| IBIS file generated by GenIBIS.pl Version 3.28
|   awr1642_q1_3v3_fcbga161
[IBIS ver]   4.1
[File name]   awr1642_q1_3v3_fcbga161.ibs
[File Rev]   1.1
[Date]   Mon Mar 13, 2017, 18:0:35
[Source]   Data created at Texas Instruments
[Notes]   1) NOT YET CHECKED BY IBISCK4. Once checked update notes
   section with any relevant information.
   2) Model not valid until this section updated.
   Some pins may contain selectors which are not valid options
   for that particular pin.
   Please refer to the device datasheet for information on picking
   the correct selector model, which depends on various software
   register configurations.
   Some pins are modeled as IO or tri-state for output mode.
   3) converted rev1.0 to rev1.1 by hand, part# change
[Disclaimer] Please be aware that in the absence of a written agreement,
   Texas Instruments (TI) assumes no liability for: 1) the
   accuracy of the IBIS models provided to your company, 2) the
   proper functioning of these IBIS models in your design or for
   any resulting applications, or, 3) infringement of patents,
   copyrights, or intellectual property rights resulting from
   your use of these IBIS models. TI provides IBIS models as a
   service to our customers and therefore reserves the right to
   limit distribution of the IBIS models.
[Copyright]   Property of Texas Instruments Incorporated. Unauthorised
   reproduction and/or distribution is strictly prohibited. This
   product is protected under copyright law and trade secret law
   as an unpublished work. Created 2010,(C) Copyright 2010,
   Texas Instruments Incorporated., All Rights Reserved. These
   commodities are under the U.S. Government distribution license
   control.As such,they are not to be re-exported without the
   prior approval of the U.S. Department of Commerce.
|   Component awr1642_q1_3v3_fcbga161
[Component]   awr1642_q1_3v3_fcbga161
[Manufacturer]   Texas Instruments.
| Source IO level model revisions
|Model   Revision   Date
|BC1833DV40DCPBFBP18LL_OD_FS_SSDLV  1.0   May 27, 2010
|OLVDS18_SSDHH   1.0   Nov 14, 2016
|BC1833DV40DCPBFBP18LL_SSDLV   1.0   May 27, 2010
[Package Model] awr1642_q1_3v3_fcbga161
[Package]
|   typ   min   max
R_pkg   0.147827121052632   18.2775E-3   506.793E-3
L_pkg   1.74484056140351E-009 0.245382E-9   5.35555E-9
C_pkg   7.81909035087719E-013 0.285311E-12   2.03823E-12
[Pin]   signal_name   model_name
D15   CLKM   NC
C15   CLKP   NC
P1   GPADC_1   NC
B13   GPADC_5   NC
P2   GPADC_2   NC
R2   GPADC_4   NC
P3   GPADC_3   NC
C14   GPADC_6   NC
H13   GPIO_0   Selector_3
J13   GPIO_1   Selector_3
K13   GPIO_2   Selector_3
K14   LVDS_TXP[1]   Model_25
J14   LVDS_TXP[0]   Model_25
L15   LVDS_CLKM   Model_25
M15   LVDS_FRCLKM   Model_25
M14   LVDS_FRCLKP   Model_25
K15   LVDS_TXM[1]   Model_25
J15   LVDS_TXM[0]   Model_25
L14   LVDS_CLKP   Model_25
N8   MCU_CLKOUT   Selector_1
N7   NERROR_IN   Selector_2
N6   NERROR_OUT   Selector_5
R3   NRESET   NC
A14   OSC_CLKOUT   NC
P9   PMIC_CLKOUT   Selector_1
N12   QSPI[1]   Selector_3
R14   QSPI[2]   Selector_3
R12   QSPI_CLK   Selector_1
R13   QSPI[0]   Selector_3
P12   QSPI[3]   Selector_3
P11   QSPI_CS_N   Selector_1
N4   RS232_RX   Selector_6
N5   RS232_TX   Selector_1
M2   RX1   NC
K2   RX2   NC
H2   RX3   NC
F2   RX4   NC
P13   SPI_HOST_INTR   Selector_1
E14   SPIA_MISO   Selector_1
D13   SPIA_MOSI   Selector_6
C13   SPIA_CS_N   Selector_6
E13   SPIA_CLK   Selector_6
F13   SPIB_MOSI   Selector_6
H14   SPIB_CS_N   Selector_6
G14   SPIB_MISO   Selector_1
F14   SPIB_CLK   Selector_6
P4   SYNC_IN   Selector_6
G13   SYNC_OUT   Selector_1
P10   TCK   Selector_6
R11   TDI   Selector_6
N13   TDO   Selector_1
N10   TMS   Selector_6
B8   TRACE_DATA_14   Selector_6
N15   TRACE_CLK   Selector_6
C9   TRACE_DATA_11   Selector_6
P6   TRACE_DATA_3   Selector_6
P5   TRACE_DATA_1   Selector_6
C8   TRACE_DATA_12   Selector_6
B14   TRACE_DATA_9   Selector_6
R4   TRACE_DATA_0   Selector_6
P8   TRACE_DATA_7   Selector_6
P7   TRACE_DATA_5   Selector_6
R5   TRACE_DATA_2   Selector_6
N14   TRACE_CTL   Selector_6
A9   TRACE_DATA_15   Selector_6
R8   TRACE_DATA_6   Selector_6
R7   TRACE_DATA_4   Selector_6
B9   TRACE_DATA_13   Selector_6
B15   TRACE_DATA_10   Selector_6
D14   TRACE_DATA_8   Selector_6
B4   TX1   NC
B6   TX2   NC
B10   VBGAP   NC
H15   VDDIN   NC
N11   VDDIN   NC
P15   VDDIN   NC
R6   VDDIN   NC
C2   VIN_13RF2   NC
D2   VIN_13RF2   NC
F5   VIN_18BB   NC
K5   VIN_18BB   NC
B12   VIN_18VCO   NC
G5   VIN_13RF1   NC
H5   VIN_13RF1   NC
J5   VIN_13RF1   NC
B11   VIN_18CLK   NC
G15   VIN_SRAM   NC
R9   VIOIN_18   NC
F15   VIOIN   NC
R10   VIOIN   NC
E15   VIOIN_18DIFF   NC
P14   VNWA   NC
A10   VOUT_14APLL1   NC
A2   VOUT_PA   NC
B2   VOUT_PA   NC
A13   VOUT_14SYNTH   NC
L13   VPP   NC
E10   VSS   NC
E11   VSS   NC
E5   VSS   NC
E6   VSS   NC
E8   VSS   NC
F11   VSS   NC
F9   VSS   NC
G10   VSS   NC
G6   VSS   NC
G7   VSS   NC
G8   VSS   NC
H11   VSS   NC
H7   VSS   NC
H9   VSS   NC
J10   VSS   NC
J6   VSS   NC
J7   VSS   NC
J8   VSS   NC
K10   VSS   NC
K11   VSS   NC
K7   VSS   NC
K8   VSS   NC
K9   VSS   NC
L10   VSS   NC
L5   VSS   NC
L6   VSS   NC
L8   VSS   NC
R15   VSS   NC
A1   VSSA   NC
A15   VSSA   NC
A3   VSSA   NC
A5   VSSA   NC
A7   VSSA   NC
B1   VSSA   NC
B3   VSSA   NC
B5   VSSA   NC
B7   VSSA   NC
C1   VSSA   NC
C3   VSSA   NC
C4   VSSA   NC
C5   VSSA   NC
C6   VSSA   NC
C7   VSSA   NC
E1   VSSA   NC
E2   VSSA   NC
E3   VSSA   NC
F3   VSSA   NC
G1   VSSA   NC
G2   VSSA   NC
G3   VSSA   NC
H3   VSSA   NC
J1   VSSA   NC
J2   VSSA   NC
J3   VSSA   NC
K3   VSSA   NC
L1   VSSA   NC
L2   VSSA   NC
L3   VSSA   NC
M3   VSSA   NC
N1   VSSA   NC
N2   VSSA   NC
N3   VSSA   NC
R1   VSSA   NC
N9   WARM_RESET   Selector_4
[Diff Pin] inv_pin  vdiff  tdelay_typ
|Differential signal data for cell OLVDS18_SSDHH
|LVDS_TXM[1]   LVDS_TXP[1]
K15   K14   200m   NA
|LVDS_TXM[0]   LVDS_TXP[0]
J15   J14   200m   NA
|LVDS_CLKM   LVDS_CLKP
L15   L14   200m   NA
|LVDS_FRCLKM   LVDS_FRCLKP
M15   M14   200m   NA
|   Usage OUTPUT#3.3#X#X#BC1833DV40DCPBFBP18LL_SSDLV.PAD
|   Base model BC1833DV40DCPBFBP18LL_SSDLV
[Model Selector] Selector_1
Model_10 I/O,3.3V,WEAK_PU_ON,FAST,IND,5%,BC40D_V_PU_ON_5P_!SC1_3P3
Model_11 I/O,3.3V,WEAK_PUPDOFF,FAST,IND,5%,BC40D_V_PUPDOFF_5P_!SC1_3P3
Model_12 I/O,3.3V,WEAK_PU_ON,SLOW,IND,5%,BC40D_V_PU_ON_5P_SC1_3P3
Model_19 I/O,3.3V,WEAK_PUPDOFF,SLOW,IND,10%,BC40D_V_PUPDOFF_10P_SC1_3P3
Model_20 I/O,3.3V,WEAK_PD_ON,FAST,IND,10%,BC40D_V_PD_ON_10P_!SC1_3P3
Model_21 I/O,3.3V,WEAK_PD_ON,SLOW,IND,10%,BC40D_V_PD_ON_10P_SC1_3P3
Model_22 I/O,3.3V,WEAK_PU_ON,FAST,IND,10%,BC40D_V_PU_ON_10P_!SC1_3P3
Model_23 I/O,3.3V,WEAK_PUPDOFF,FAST,IND,10%,BC40D_V_PUPDOFF_10P_!SC1_3P3
Model_24 I/O,3.3V,WEAK_PU_ON,SLOW,IND,10%,BC40D_V_PU_ON_10P_SC1_3P3
Model_7 I/O,3.3V,WEAK_PUPDOFF,SLOW,IND,5%,BC40D_V_PUPDOFF_5P_SC1_3P3
Model_8 I/O,3.3V,WEAK_PD_ON,FAST,IND,5%,BC40D_V_PD_ON_5P_!SC1_3P3
Model_9 I/O,3.3V,WEAK_PD_ON,SLOW,IND,5%,BC40D_V_PD_ON_5P_SC1_3P3
|   Usage INPUT#3.3#X#X#BC1833DV40DCPBFBP18LL_OD_FS_SSDLV.PAD
|   Base model BC1833DV40DCPBFBP18LL_OD_FS_SSDLV
[Model Selector] Selector_2
Model_32 I/O_OPEN_DRAIN,3.3V,WEAK_PUPDOFF,SLOW,IND,5%,BC40D_V_PUPDOFF_5P_SC1_3P
Model_33 I/O_OPEN_DRAIN,3.3V,WEAK_PD_ON,FAST,IND,5%,BC40D_V_PD_ON_5P_!SC1_3P3
Model_34 I/O_OPEN_DRAIN,3.3V,WEAK_PD_ON,SLOW,IND,5%,BC40D_V_PD_ON_5P_SC1_3P3
Model_35 I/O_OPEN_DRAIN,3.3V,WEAK_PU_ON,FAST,IND,5%,BC40D_V_PU_ON_5P_!SC1_3P3
Model_36 I/O_OPEN_DRAIN,3.3V,WEAK_PUPDOFF,FAST,IND,5%,BC40D_V_PUPDOFF_5P_!SC1_3
Model_37 I/O_OPEN_DRAIN,3.3V,WEAK_PU_ON,SLOW,IND,5%,BC40D_V_PU_ON_5P_SC1_3P3
Model_44 I/O_OPEN_DRAIN,3.3V,WEAK_PUPDOFF,SLOW,IND,10%,BC40D_V_PUPDOFF_10P_SC1_
Model_45 I/O_OPEN_DRAIN,3.3V,WEAK_PD_ON,FAST,IND,10%,BC40D_V_PD_ON_10P_!SC1_3P3
Model_46 I/O_OPEN_DRAIN,3.3V,WEAK_PD_ON,SLOW,IND,10%,BC40D_V_PD_ON_10P_SC1_3P3
Model_47 I/O_OPEN_DRAIN,3.3V,WEAK_PU_ON,FAST,IND,10%,BC40D_V_PU_ON_10P_!SC1_3P3
Model_48 I/O_OPEN_DRAIN,3.3V,WEAK_PUPDOFF,FAST,IND,10%,BC40D_V_PUPDOFF_10P_!SC1
Model_49 I/O_OPEN_DRAIN,3.3V,WEAK_PU_ON,SLOW,IND,10%,BC40D_V_PU_ON_10P_SC1_3P3
|   Usage I/O#3.3#X#X#BC1833DV40DCPBFBP18LL_SSDLV.PAD
|   Base model BC1833DV40DCPBFBP18LL_SSDLV
[Model Selector] Selector_3
Model_10 I/O,3.3V,WEAK_PU_ON,FAST,IND,5%,BC40D_V_PU_ON_5P_!SC1_3P3
Model_11 I/O,3.3V,WEAK_PUPDOFF,FAST,IND,5%,BC40D_V_PUPDOFF_5P_!SC1_3P3
Model_12 I/O,3.3V,WEAK_PU_ON,SLOW,IND,5%,BC40D_V_PU_ON_5P_SC1_3P3
Model_19 I/O,3.3V,WEAK_PUPDOFF,SLOW,IND,10%,BC40D_V_PUPDOFF_10P_SC1_3P3
Model_20 I/O,3.3V,WEAK_PD_ON,FAST,IND,10%,BC40D_V_PD_ON_10P_!SC1_3P3
Model_21 I/O,3.3V,WEAK_PD_ON,SLOW,IND,10%,BC40D_V_PD_ON_10P_SC1_3P3
Model_22 I/O,3.3V,WEAK_PU_ON,FAST,IND,10%,BC40D_V_PU_ON_10P_!SC1_3P3
Model_23 I/O,3.3V,WEAK_PUPDOFF,FAST,IND,10%,BC40D_V_PUPDOFF_10P_!SC1_3P3
Model_24 I/O,3.3V,WEAK_PU_ON,SLOW,IND,10%,BC40D_V_PU_ON_10P_SC1_3P3
Model_7 I/O,3.3V,WEAK_PUPDOFF,SLOW,IND,5%,BC40D_V_PUPDOFF_5P_SC1_3P3
Model_8 I/O,3.3V,WEAK_PD_ON,FAST,IND,5%,BC40D_V_PD_ON_5P_!SC1_3P3
Model_9 I/O,3.3V,WEAK_PD_ON,SLOW,IND,5%,BC40D_V_PD_ON_5P_SC1_3P3
|   Usage I/O#3.3#X#X#BC1833DV40DCPBFBP18LL_OD_FS_SSDLV.PAD
|   Base model BC1833DV40DCPBFBP18LL_OD_FS_SSDLV
[Model Selector] Selector_4
Model_32 I/O_OPEN_DRAIN,3.3V,WEAK_PUPDOFF,SLOW,IND,5%,BC40D_V_PUPDOFF_5P_SC1_3P
Model_33 I/O_OPEN_DRAIN,3.3V,WEAK_PD_ON,FAST,IND,5%,BC40D_V_PD_ON_5P_!SC1_3P3
Model_34 I/O_OPEN_DRAIN,3.3V,WEAK_PD_ON,SLOW,IND,5%,BC40D_V_PD_ON_5P_SC1_3P3
Model_35 I/O_OPEN_DRAIN,3.3V,WEAK_PU_ON,FAST,IND,5%,BC40D_V_PU_ON_5P_!SC1_3P3
Model_36 I/O_OPEN_DRAIN,3.3V,WEAK_PUPDOFF,FAST,IND,5%,BC40D_V_PUPDOFF_5P_!SC1_3
Model_37 I/O_OPEN_DRAIN,3.3V,WEAK_PU_ON,SLOW,IND,5%,BC40D_V_PU_ON_5P_SC1_3P3
Model_44 I/O_OPEN_DRAIN,3.3V,WEAK_PUPDOFF,SLOW,IND,10%,BC40D_V_PUPDOFF_10P_SC1_
Model_45 I/O_OPEN_DRAIN,3.3V,WEAK_PD_ON,FAST,IND,10%,BC40D_V_PD_ON_10P_!SC1_3P3
Model_46 I/O_OPEN_DRAIN,3.3V,WEAK_PD_ON,SLOW,IND,10%,BC40D_V_PD_ON_10P_SC1_3P3
Model_47 I/O_OPEN_DRAIN,3.3V,WEAK_PU_ON,FAST,IND,10%,BC40D_V_PU_ON_10P_!SC1_3P3
Model_48 I/O_OPEN_DRAIN,3.3V,WEAK_PUPDOFF,FAST,IND,10%,BC40D_V_PUPDOFF_10P_!SC1
Model_49 I/O_OPEN_DRAIN,3.3V,WEAK_PU_ON,SLOW,IND,10%,BC40D_V_PU_ON_10P_SC1_3P3
|   Usage OUTPUT#3.3#X#X#BC1833DV40DCPBFBP18LL_OD_FS_SSDLV.PAD
|   Base model BC1833DV40DCPBFBP18LL_OD_FS_SSDLV
[Model Selector] Selector_5
Model_32 I/O_OPEN_DRAIN,3.3V,WEAK_PUPDOFF,SLOW,IND,5%,BC40D_V_PUPDOFF_5P_SC1_3P
Model_33 I/O_OPEN_DRAIN,3.3V,WEAK_PD_ON,FAST,IND,5%,BC40D_V_PD_ON_5P_!SC1_3P3
Model_34 I/O_OPEN_DRAIN,3.3V,WEAK_PD_ON,SLOW,IND,5%,BC40D_V_PD_ON_5P_SC1_3P3
Model_35 I/O_OPEN_DRAIN,3.3V,WEAK_PU_ON,FAST,IND,5%,BC40D_V_PU_ON_5P_!SC1_3P3
Model_36 I/O_OPEN_DRAIN,3.3V,WEAK_PUPDOFF,FAST,IND,5%,BC40D_V_PUPDOFF_5P_!SC1_3
Model_37 I/O_OPEN_DRAIN,3.3V,WEAK_PU_ON,SLOW,IND,5%,BC40D_V_PU_ON_5P_SC1_3P3
Model_44 I/O_OPEN_DRAIN,3.3V,WEAK_PUPDOFF,SLOW,IND,10%,BC40D_V_PUPDOFF_10P_SC1_
Model_45 I/O_OPEN_DRAIN,3.3V,WEAK_PD_ON,FAST,IND,10%,BC40D_V_PD_ON_10P_!SC1_3P3
Model_46 I/O_OPEN_DRAIN,3.3V,WEAK_PD_ON,SLOW,IND,10%,BC40D_V_PD_ON_10P_SC1_3P3
Model_47 I/O_OPEN_DRAIN,3.3V,WEAK_PU_ON,FAST,IND,10%,BC40D_V_PU_ON_10P_!SC1_3P3
Model_48 I/O_OPEN_DRAIN,3.3V,WEAK_PUPDOFF,FAST,IND,10%,BC40D_V_PUPDOFF_10P_!SC1
Model_49 I/O_OPEN_DRAIN,3.3V,WEAK_PU_ON,SLOW,IND,10%,BC40D_V_PU_ON_10P_SC1_3P3
|   Usage INPUT#3.3#X#X#BC1833DV40DCPBFBP18LL_SSDLV.PAD
|   Base model BC1833DV40DCPBFBP18LL_SSDLV
[Model Selector] Selector_6
Model_10 I/O,3.3V,WEAK_PU_ON,FAST,IND,5%,BC40D_V_PU_ON_5P_!SC1_3P3
Model_11 I/O,3.3V,WEAK_PUPDOFF,FAST,IND,5%,BC40D_V_PUPDOFF_5P_!SC1_3P3
Model_12 I/O,3.3V,WEAK_PU_ON,SLOW,IND,5%,BC40D_V_PU_ON_5P_SC1_3P3
Model_19 I/O,3.3V,WEAK_PUPDOFF,SLOW,IND,10%,BC40D_V_PUPDOFF_10P_SC1_3P3
Model_20 I/O,3.3V,WEAK_PD_ON,FAST,IND,10%,BC40D_V_PD_ON_10P_!SC1_3P3
Model_21 I/O,3.3V,WEAK_PD_ON,SLOW,IND,10%,BC40D_V_PD_ON_10P_SC1_3P3
Model_22 I/O,3.3V,WEAK_PU_ON,FAST,IND,10%,BC40D_V_PU_ON_10P_!SC1_3P3
Model_23 I/O,3.3V,WEAK_PUPDOFF,FAST,IND,10%,BC40D_V_PUPDOFF_10P_!SC1_3P3
Model_24 I/O,3.3V,WEAK_PU_ON,SLOW,IND,10%,BC40D_V_PU_ON_10P_SC1_3P3
Model_7 I/O,3.3V,WEAK_PUPDOFF,SLOW,IND,5%,BC40D_V_PUPDOFF_5P_SC1_3P3
Model_8 I/O,3.3V,WEAK_PD_ON,FAST,IND,5%,BC40D_V_PD_ON_5P_!SC1_3P3
Model_9 I/O,3.3V,WEAK_PD_ON,SLOW,IND,5%,BC40D_V_PD_ON_5P_SC1_3P3
| Package model definition
[Define Package Model]  awr1642_q1_3v3_fcbga161
[Manufacturer]   Texas Instruments.
[OEM]   Texas Instruments.
[Description]   awr1642_q1_3v3_fcbga161 package model generated by GenIBIS.pl
[Number Of Pins]   57
[Pin Numbers]
H13   | 1 GPIO_0   I/O
J13   | 2 GPIO_1   I/O
K13   | 3 GPIO_2   I/O
K14   | 4 LVDS_TXP[1]   OUTPUT
J14   | 5 LVDS_TXP[0]   OUTPUT
L15   | 6 LVDS_CLKM   OUTPUT
M15   | 7 LVDS_FRCLKM   OUTPUT
M14   | 8 LVDS_FRCLKP   OUTPUT
K15   | 9 LVDS_TXM[1]   OUTPUT
J15   | 10 LVDS_TXM[0]   OUTPUT
L14   | 11 LVDS_CLKP   OUTPUT
N8   | 12 MCU_CLKOUT   OUTPUT
N7   | 13 NERROR_IN   INPUT
N6   | 14 NERROR_OUT   OUTPUT
P9   | 15 PMIC_CLKOUT   OUTPUT
N12   | 16 QSPI[1]   I/O
R14   | 17 QSPI[2]   I/O
R12   | 18 QSPI_CLK   OUTPUT
R13   | 19 QSPI[0]   I/O
P12   | 20 QSPI[3]   I/O
P11   | 21 QSPI_CS_N   OUTPUT
N4   | 22 RS232_RX   INPUT
N5   | 23 RS232_TX   OUTPUT
P13   | 24 SPI_HOST_INTR   OUTPUT
E14   | 25 SPIA_MISO   OUTPUT
D13   | 26 SPIA_MOSI   INPUT
C13   | 27 SPIA_CS_N   INPUT
E13   | 28 SPIA_CLK   INPUT
F13   | 29 SPIB_MOSI   INPUT
H14   | 30 SPIB_CS_N   INPUT
G14   | 31 SPIB_MISO   OUTPUT
F14   | 32 SPIB_CLK   INPUT
P4   | 33 SYNC_IN   INPUT
G13   | 34 SYNC_OUT   OUTPUT
P10   | 35 TCK   INPUT
R11   | 36 TDI   INPUT
N13   | 37 TDO   OUTPUT
N10   | 38 TMS   INPUT
B8   | 39 TRACE_DATA_14   INPUT
N15   | 40 TRACE_CLK   INPUT
C9   | 41 TRACE_DATA_11   INPUT
P6   | 42 TRACE_DATA_3   INPUT
P5   | 43 TRACE_DATA_1   INPUT
C8   | 44 TRACE_DATA_12   INPUT
B14   | 45 TRACE_DATA_9   INPUT
R4   | 46 TRACE_DATA_0   INPUT
P8   | 47 TRACE_DATA_7   INPUT
P7   | 48 TRACE_DATA_5   INPUT
R5   | 49 TRACE_DATA_2   INPUT
N14   | 50 TRACE_CTL   INPUT
A9   | 51 TRACE_DATA_15   INPUT
R8   | 52 TRACE_DATA_6   INPUT
R7   | 53 TRACE_DATA_4   INPUT
B9   | 54 TRACE_DATA_13   INPUT
B15   | 55 TRACE_DATA_10   INPUT
D14   | 56 TRACE_DATA_8   INPUT
N9   | 57 WARM_RESET   I/O
[Model Data]
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[End Model Data]
[End Package Model]
| Models and submodels in the file (25): Model_7 (I/O), Model_8 (I/O), Model_9 (I/O), Model_10 (I/O), Model_11 (I/O), Model_12 (I/O), Model_19 (I/O), Model_20 (I/O), Model_21 (I/O), Model_22 (I/O), Model_23 (I/O), Model_24 (I/O), Model_25 (Output), Model_32 (I/O_open_drain), Model_33 (I/O_open_drain), Model_34 (I/O_open_drain), Model_35 (I/O_open_drain), Model_36 (I/O_open_drain), Model_37 (I/O_open_drain), Model_44 (I/O_open_drain), Model_45 (I/O_open_drain), Model_46 (I/O_open_drain), Model_47 (I/O_open_drain), Model_48 (I/O_open_drain), Model_49 (I/O_open_drain)
